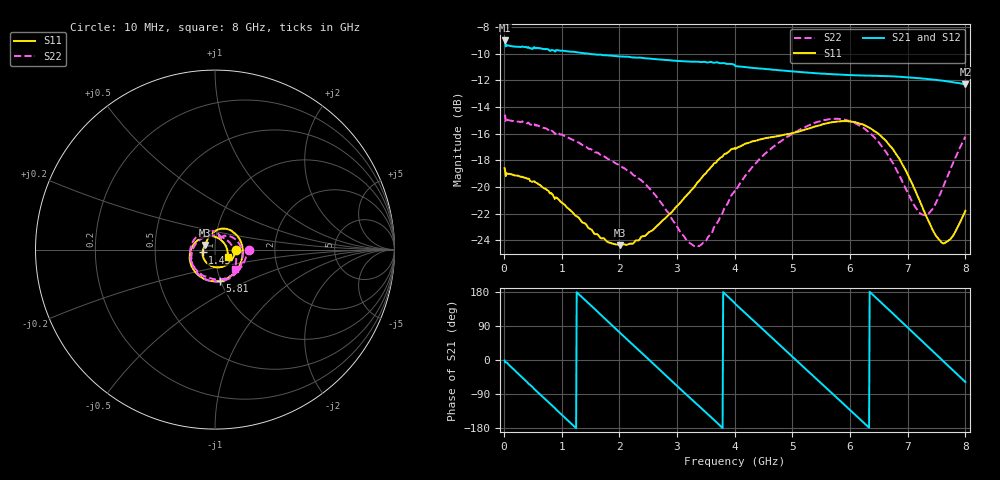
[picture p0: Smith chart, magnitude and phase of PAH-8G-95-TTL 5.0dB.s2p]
! MTS Systemtechnik GmbH
! S-Parameters
! Model: PAH-8G/95-TTL
! Attenuation Step: 5.0dB
! Rohde & Schwarz ZVB8 2Ports - Version 4.11 - 1145.1010k08 SN: 100119
! S2P File Measurements:
! S11 S21 S12 S22
# HZ  S  DB  R  50.00
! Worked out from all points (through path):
!   800 points, 10 MHz to 8 GHz, reference 50 ohm
!   highest |S21| = -9.00 dB at 10 MHz (marker M1); lowest = -12.3 dB at 8 GHz (marker M2)
!   group delay of S21, straight-line fit = 394 ps
!   lowest |S11| = -24.4 dB at 2.01 GHz (marker M3), VSWR 1.13, Z = 44.8 + j2.35 ohm
!   |S11| at or under -10 dB: start of sweep to end of sweep
!   |S22| runs from -24.4 to -14.6 dB; largest |S21 - S12| = 0.0047
!   S11 on the Smith chart (normalised r, x): 10 MHz: 1.27, -0.01; 1.45 GHz: 0.87, -0.03; 5.81 GHz: 0.99, -0.36; 8 GHz: 1.15, -0.09
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1e7  -18.59 -2.2  -9.00 -1.2  -8.90 -1.0  -14.57 -1.3
3.5e8  -19.28 -43.7  -9.50 -51.1  -9.51 -51.1  -15.14 -43.9
6.4e8  -19.91 -79.1  -9.60 -92.9  -9.58 -92.9  -15.48 -79.7
1.03e9  -21.26 -124.8  -9.78 -148.6  -9.77 -148.6  -16.12 -126.3
1.35e9  -22.63 -158.2  -9.94 165.8  -9.93 165.9  -16.83 -162.4
1.45e9  -23.00 -167.3  -9.98 151.8  -9.98 151.8  -17.09 -173.1
2.01e9  -24.35 154.4  -10.19 71.9  -10.21 72.1  -18.40 131.1
2.37e9  -23.80 137.9  -10.29 21.3  -10.29 21.4  -19.47 101.3
2.68e9  -22.82 123.4  -10.42 -23.0  -10.42 -22.8  -20.94 78.5
3.27e9  -20.14 93.7  -10.60 -106.4  -10.62 -106.8  -24.36 60.3
3.67e9  -18.19 70.2  -10.65 -162.3  -10.63 -161.8  -22.85 64.3
4.01e9  -17.15 45.7  -10.93 148.2  -10.92 148.1  -20.33 52.0
4.56e9  -16.32 8.1  -11.15 70.6  -11.17 70.6  -17.39 18.1
4.96e9  -16.01 -18.3  -11.31 14.1  -11.32 14.0  -16.12 -10.8
5.34e9  -15.54 -43.9  -11.44 -39.1  -11.46 -39.1  -15.29 -39.8
5.81e9  -15.08 -80.8  -11.56 -105.1  -11.59 -105.2  -14.89 -79.8
6.26e9  -15.39 -123.0  -11.64 -168.8  -11.65 -168.8  -15.66 -124.3
6.67e9  -16.81 -166.7  -11.69 132.9  -11.69 133.0  -17.70 -172.1
6.99e9  -18.97 155.0  -11.77 87.0  -11.77 87.1  -20.35 139.9
7.32e9  -22.16 104.8  -11.89 39.6  -11.88 39.6  -22.12 70.5
7.63e9  -24.22 40.8  -12.04 -4.9  -12.04 -5.0  -19.81 6.6
8e9  -21.79 -30.3  -12.30 -58.2  -12.30 -58.2  -16.22 -45.1
